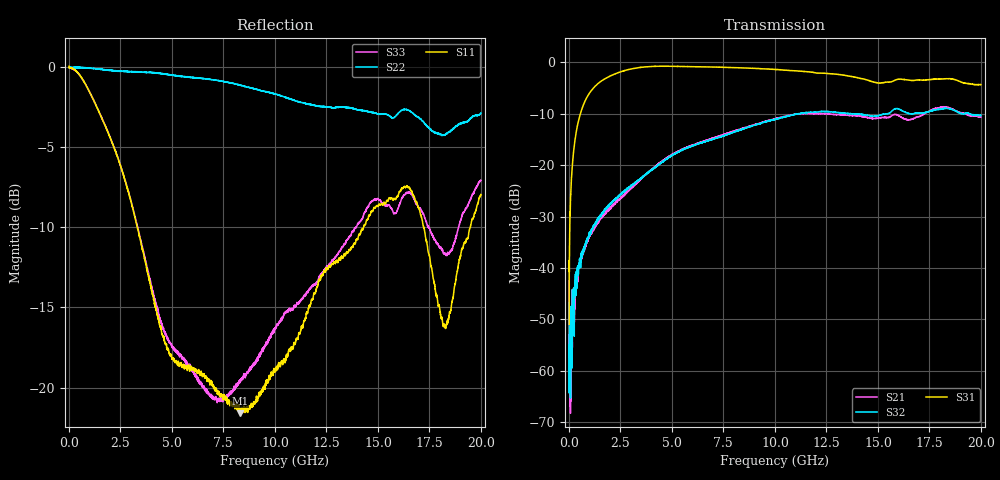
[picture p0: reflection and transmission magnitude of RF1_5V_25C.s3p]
!Keysight Technologies,N5244B,MY57181157,A.18.40.03
!Date: Friday, December 19, 2025 13:28:31
!Correction: S11(C  3-Port  )
!S12(C  3-Port  )
!S13(C  3-Port  )
!S21(C  3-Port  )
!S22(C  3-Port  )
!S23(C  3-Port  )
!S31(C  3-Port  )
!S32(C  3-Port  )
!S33(C  3-Port  )
!S3P File: Measurements: <S11,S12,S13>,
!<S21,S22,S23>,
!<S31,S32,S33>:
# Hz S  dB  R 50
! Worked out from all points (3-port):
!   3999 points, 10 MHz to 20 GHz, reference 50 ohm
!   strongest paths, dB at 10 MHz, 5.005 GHz, 10.01 GHz, 15.01 GHz, 20 GHz:
!     S31: -51.0, -0.8, -1.4, -4.0, -4.3
!     S32: -46.7, -18.1, -11.2, -10.4, -10.3
!     S21: -42.5, -17.9, -11.0, -10.8, -10.7
!   lowest |S11| = -21.6 dB at 8.295 GHz (marker M1), VSWR 1.18, Z = 46.2 - j7.04 ohm
!   |S11| at or under -10 dB: 3.32 GHz to 14.3 GHz (10.98 GHz wide, 125 % of centre); 17.23 GHz to 19.48 GHz (2.257 GHz wide, 12.3 % of centre)
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1e7  0.06 -0.6  -51.18 112.7  -56.38 -174.5
     -42.53 -88.6  -0.03 -0.2  -43.40 -58.8
     -51.02 127.2  -46.75 -93.4  -0.01 -0.6
1.15e8  -0.06 -5.0  -49.74 94.0  -23.32 90.6
        -50.50 66.1  -0.04 -1.2  -46.92 88.5
        -23.23 90.7  -57.05 49.2  -0.07 -4.9
2.55e8  -0.14 -10.9  -44.98 103.5  -16.46 81.0
        -45.82 102.1  -0.03 -2.5  -44.13 115.0
        -16.45 81.1  -43.89 107.7  -0.16 -10.7
1.09e9  -1.78 -41.1  -33.10 83.1  -5.50 48.5
        -33.24 82.9  -0.07 -9.7  -33.08 81.4
        -5.49 48.5  -32.96 83.6  -1.78 -39.4
3.675e9  -12.02 -77.8  -22.05 78.4  -0.92 0.9
         -22.03 79.3  -0.32 -21.1  -22.04 70.2
         -0.91 0.9  -22.00 70.2  -11.83 -90.7
8.295e9  -21.61 -114.3  -13.08 34.1  -1.08 -42.3
         -13.04 34.2  -1.11 -69.1  -13.17 27.4
         -1.08 -42.4  -13.24 27.3  -19.68 -171.8
1.0005e10  -19.00 -145.5  -11.02 15.4  -1.40 -55.6
           -11.01 15.5  -1.67 -92.9  -11.11 8.4
           -1.39 -55.6  -11.17 8.5  -16.38 170.0
1.4335e10  -9.86 149.3  -10.63 -37.9  -3.29 -86.8
           -10.62 -37.9  -2.70 -177.5  -10.23 -44.5
           -3.29 -86.8  -10.20 -44.4  -9.10 149.7
1.8255e10  -16.19 115.7  -8.70 -73.4  -3.21 -105.4
           -8.69 -73.3  -4.22 114.9  -8.96 -80.7
           -3.23 -105.4  -8.96 -80.6  -11.64 116.0
2e10  -7.96 107.5  -10.71 -96.2  -4.34 -117.4
      -10.67 -96.0  -2.86 93.0  -10.35 -99.3
      -4.35 -117.2  -10.34 -99.5  -7.05 135.8
